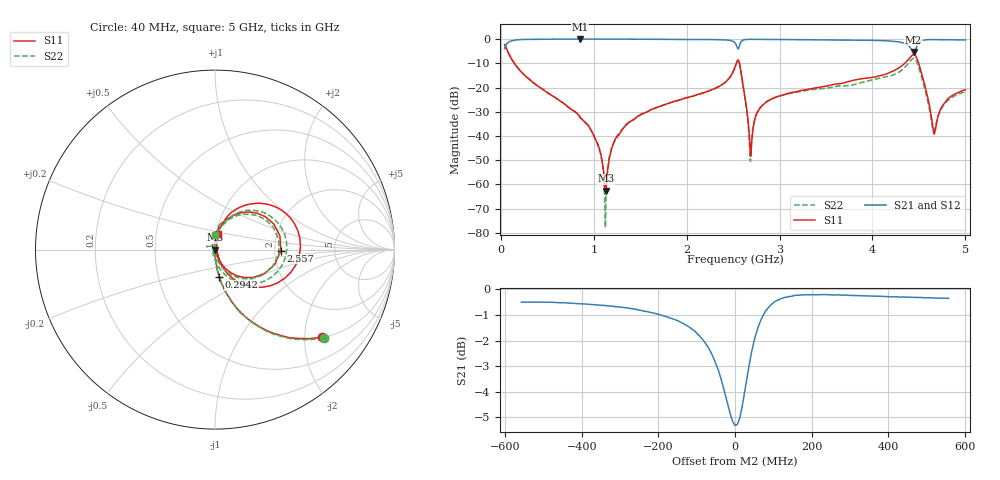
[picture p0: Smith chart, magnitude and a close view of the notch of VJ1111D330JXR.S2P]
! VJ1111D330JXR
! DATE 02/16/2022  10:25
! CAPACITORS MOUNTED IN SERIES ON 25 MIL THICK MICROSTRIP SUBSTRATE
# GHz  S  MA  R  50.00
!  FREQ  S11M  S11A  S21M  S21A  S12M  S12A  S22M  S22A
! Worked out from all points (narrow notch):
!   801 points, 40 MHz to 5 GHz, reference 50 ohm
!   highest |S21| = -0.01 dB at 852.2 MHz (marker M1); lowest = -5.3 dB at 4.442 GHz (marker M2)
!   notch at M2: 5.1 dB deep, 93.4 MHz wide at half that depth
!   lowest |S11| = -62.6 dB at 1.131 GHz (marker M3), VSWR 1.00, Z = 50.1 + j0.029 ohm
!   |S11| at or under -10 dB: 143.8 MHz to 2.534 GHz (2.39 GHz wide, 179 % of centre); 2.568 GHz to 4.347 GHz (1.779 GHz wide, 51.5 % of centre); 4.497 GHz to end of sweep
!   |S22| runs from -77.9 to -2.1 dB; largest |S21 - S12| = 0.039
!   S11 on the Smith chart (normalised r, x): 40 MHz: 1.01, -2.43; 294.2 MHz: 1.00, -0.31; 2.557 GHz: 2.15, -0.03; 5 GHz: 1.02, +0.18
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0.04  0.7704 -39.4  0.6353 50.7  0.6326 50.7  0.7807 -39.1
0.1268  0.3541 -69.3  0.9236 20.5  0.9465 21.5  0.3599 -69.2
0.2942  0.1542 -81.3  0.9872 9.2  0.9935 8.9  0.1548 -81.5
0.8522  0.02427 -89.3  0.999 2.6  1.004 2.4  0.02451 -88.0
0.8708  0.0225 -87.5  0.998 2.4  1.003 2.3  0.02235 -87.6
1.0444  0.00663 -83.8  0.9965 1.7  1.003 1.5  0.006648 -86.3
1.1312  0.0007408 23.0  0.9967 1.5  1.003 1.3  0.0005466 58.6
1.187  0.004884 81.5  0.9966 1.3  1.003 1.1  0.005239 84.6
1.28  0.01136 83.9  0.9959 1.0  1.002 0.8  0.01184 89.1
1.6954  0.03989 85.8  0.9914 -0.0  0.9974 -0.2  0.03961 86.2
2.334  0.1018 80.0  0.9722 -2.7  0.9774 -2.9  0.1015 78.9
2.52  0.265 51.8  0.8364 -10.1  0.8416 -10.3  0.2592 49.7
2.5572  0.3662 -0.8  0.632 6.3  0.6358 6.1  0.3561 -3.9
2.6874  0.003773 -3.2  0.9869 3.4  0.9927 3.2  0.002987 150.8
2.83  0.04522 86.3  0.984 1.0  0.9899 0.8  0.04626 92.5
3.3508  0.09518 82.2  0.967 -1.4  0.9727 -1.5  0.09047 84.7
4.1754  0.1995 69.1  0.916 -5.8  0.9223 -6.0  0.171 69.2
4.442  0.4771 7.5  0.5426 3.5  0.5457 3.3  0.4008 6.2
4.4978  0.3121 -42.4  0.8231 20.2  0.8283 20.0  0.2607 -47.4
4.6652  0.01091 9.1  0.9766 4.7  0.9823 4.6  0.0129 171.3
4.783  0.05016 76.2  0.9713 2.1  0.9769 1.9  0.04779 104.0
5  0.0898 77.5  0.9605 -0.1  0.9651 -0.2  0.08178 91.9
